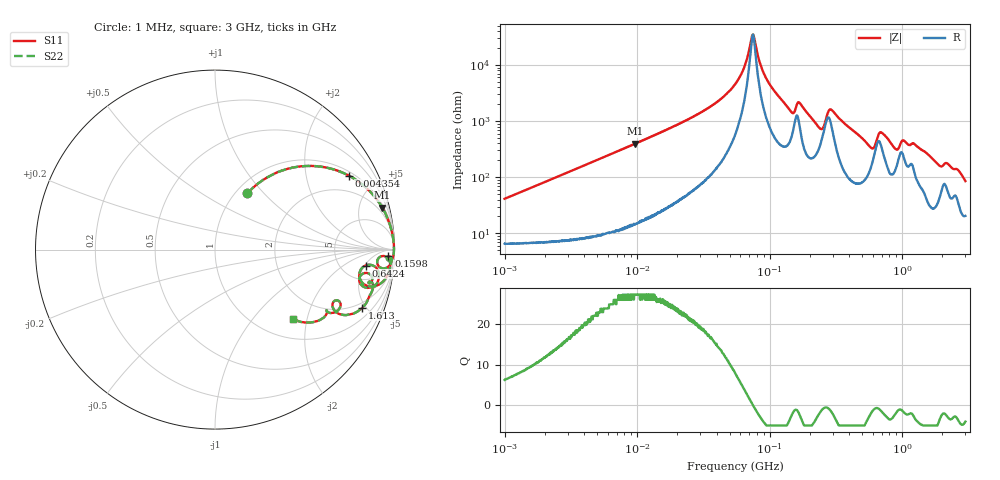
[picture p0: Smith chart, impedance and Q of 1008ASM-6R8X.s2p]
!s-Parameter Generated by FASTRON Sdn. Bhd.
!FASTRON P/N : 1008ASM-6R8X
!Keysight Technologies: E4991B_MY54100416_A.01.15
!Date: Wed Jun 19 15:39:53 2024
!Version  :Rev00  Wed Jun 19 15:39:53 2024
!Data & Calibration Information:
!Freq  S11  S21  S12  S22
!PortZ  Port1:50+j0  Port2:50+j0
!When reading reference impedance value at option line is always used.
! Remarks : This data is being provided solely for informational purposes.
# Hz S dB R 50
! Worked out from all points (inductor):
!   1601 points, 1 MHz to 3 GHz, reference 50 ohm
!   read as one part in series: L = 6.47 uH near 1.041 MHz
!   highest Q = 27.3 at 9.649 MHz (marker M1), where L = 6.53 uH
!   self-resonance near 74.7 MHz
!   S11 on the Smith chart (normalised r, x): 1 MHz: 1.13, +0.81; 4.354 MHz: 1.17, +3.53; 159.8 MHz: 26, -29; 642.4 MHz: 8.52, -5.23; 1.613 GHz: 1.61, -4.74; 3 GHz: 1.41, -1.65
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1000000  -8.83 60.0  -1.14 -20.9  -1.14 -20.9  -8.83 60.0
3804036  -1.72 32.0  -5.50 -55.0  -5.50 -55.0  -1.72 32.0
4354327  -1.38 28.8  -6.34 -58.5  -6.34 -58.5  -1.38 28.8
9648503  -0.34 14.1  -12.30 -73.8  -12.30 -73.8  -0.34 14.1
1.447069e7  -0.17 9.4  -15.80 -78.4  -15.80 -78.4  -0.17 9.4
3.526298e7  -0.04 3.2  -25.00 -83.4  -25.00 -83.4  -0.04 3.2
5.504702e7  -0.03 1.2  -33.30 -81.5  -33.30 -81.5  -0.03 1.2
6.364388e7  -0.02 0.6  -38.70 -75.8  -38.70 -75.8  -0.02 0.6
7.507101e7  -0.02 -0.0  -50.90 4.8  -50.90 4.8  -0.02 -0.0
8.679508e7  -0.03 -0.6  -39.10 73.1  -39.10 73.1  -0.03 -0.6
1.003501e8  -0.03 -1.3  -33.10 79.0  -33.10 79.0  -0.03 -1.3
1.453231e8  -0.22 -3.6  -23.50 66.6  -23.50 66.6  -0.22 -3.6
1.59818e8  -0.30 -2.2  -26.00 47.2  -26.00 47.2  -0.30 -2.2
2.083556e8  -0.18 -5.0  -21.10 73.8  -21.10 73.8  -0.18 -5.0
2.457655e8  -0.76 -5.8  -17.90 46.5  -17.90 46.5  -0.76 -5.8
2.898922e8  -0.31 -2.8  -24.40 52.7  -24.40 52.7  -0.31 -2.8
5.63991e8  -1.02 -13.4  -12.20 56.8  -12.20 56.8  -1.02 -13.4
6.423554e8  -1.48 -6.0  -14.70 28.8  -14.70 28.8  -1.48 -6.0
6.924261e8  -0.83 -6.7  -16.80 47.6  -16.80 47.6  -0.83 -6.7
7.925923e8  -0.68 -11.2  -13.90 62.6  -13.90 62.6  -0.68 -11.2
1.613037e9  -1.08 -21.5  -8.65 61.1  -8.65 61.1  -1.08 -21.5
3e9  -4.69 -41.6  -3.29 34.5  -3.29 34.5  -4.69 -41.6
